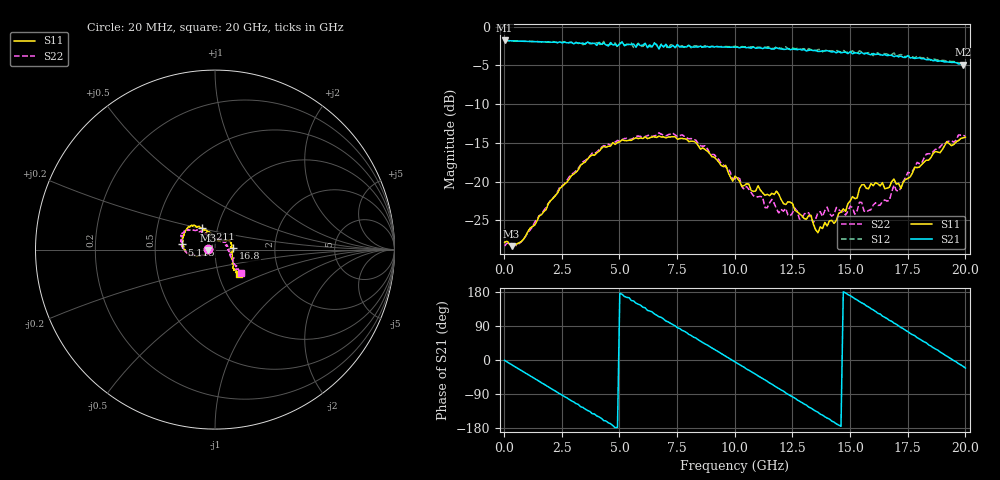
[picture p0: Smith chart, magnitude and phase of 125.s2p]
!Agilent Technologies,N5230A,US43500223,A.07.50.48
!Agilent N5230A: A.07.50.48
!Date: Saturday, September 19, 2015 18:53:34
!Correction: S11(Full 2 Port(1,2))
!S21(Full 2 Port(1,2))
!S12(Full 2 Port(1,2))
!S22(Full 2 Port(1,2))
!S2P File: Measurements: S11, S21, S12, S22:
# Hz S  dB  R 50
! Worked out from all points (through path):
!   201 points, 20 MHz to 20 GHz, reference 50 ohm
!   highest |S21| = -1.80 dB at 20 MHz (marker M1); lowest = -4.9 dB at 19.9 GHz (marker M2)
!   group delay of S21, straight-line fit = 102 ps
!   lowest |S11| = -28.3 dB at 319.7 MHz (marker M3), VSWR 1.08, Z = 46.3 - j0.164 ohm
!   |S11| at or under -10 dB: start of sweep to end of sweep
!   |S22| runs from -28.3 to -13.7 dB; largest |S21 - S12| = 0.054
!   S11 on the Smith chart (normalised r, x): 20 MHz: 0.92, +0.00; 5.115 GHz: 0.69, +0.04; 9.211 GHz: 0.84, +0.20; 16.8 GHz: 1.22, +0.02; 20 GHz: 1.26, -0.36
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2e7  -27.82 178.6  -1.80 -0.8  -1.79 -0.8  -28.28 178.6
3.197e8  -28.31 -177.4  -1.84 -12.2  -1.84 -12.1  -27.96 -177.0
1.9181e9  -22.82 -154.8  -1.96 -71.0  -1.96 -70.8  -22.79 -155.2
3.4166e9  -17.63 -166.3  -2.14 -125.1  -2.34 -124.6  -17.45 -166.9
4.3157e9  -15.46 -176.8  -2.13 -159.9  -1.92 -157.2  -15.35 -178.0
5.1149e9  -14.61 171.2  -1.97 173.4  -2.02 173.9  -14.58 173.9
6.1139e9  -14.22 156.0  -2.15 137.8  -2.26 140.4  -14.18 163.4
6.7133e9  -14.12 148.0  -2.90 114.2  -2.82 115.6  -13.71 157.2
8.012e9  -14.85 133.1  -2.44 67.3  -2.42 68.9  -14.48 146.2
9.2108e9  -17.16 121.8  -2.56 24.7  -2.58 26.1  -16.84 132.0
1.001e10  -19.28 113.1  -2.66 -5.0  -2.55 -3.3  -19.61 120.6
1.08092e10  -21.26 105.6  -2.63 -34.3  -2.61 -32.6  -21.81 110.8
1.18082e10  -21.20 101.2  -2.72 -71.7  -2.59 -69.2  -23.49 90.7
1.25075e10  -22.82 96.4  -2.90 -97.4  -2.74 -95.0  -23.99 87.2
1.34066e10  -25.47 83.7  -3.10 -130.9  -3.04 -129.9  -25.25 78.0
1.5005e10  -22.46 43.7  -3.24 169.8  -3.26 173.6  -23.16 51.3
1.67033e10  -20.72 10.6  -3.70 104.6  -3.70 107.7  -22.42 -5.9
1.68032e10  -19.99 4.2  -3.71 102.2  -3.62 104.1  -21.34 -11.2
1.76024e10  -19.40 -27.8  -4.03 70.5  -3.74 73.2  -18.87 -29.9
1.85015e10  -16.91 -46.0  -4.26 36.9  -4.34 38.7  -16.40 -37.0
1.99001e10  -14.35 -45.4  -4.90 -16.7  -4.69 -15.0  -13.99 -42.8
2e10  -14.26 -45.6  -4.87 -21.2  -4.74 -18.5  -14.18 -42.7
